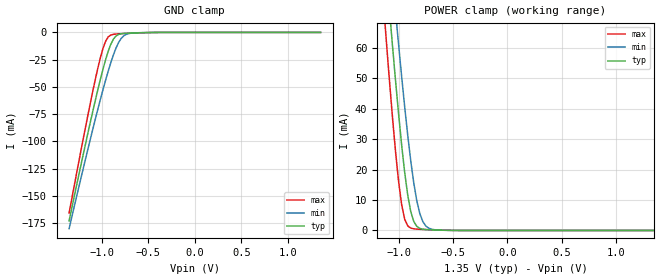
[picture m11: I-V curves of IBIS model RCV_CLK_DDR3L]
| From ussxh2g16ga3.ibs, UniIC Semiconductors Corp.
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|   Model RCV_CLK_DDR3L
[Model] RCV_CLK_DDR3L
Model_type Input
Vinl =  0.540V
Vinh =  0.810V
C_comp   0.694pF   0.694pF   0.694pF
[Model Spec]
Vinh   0.810V   0.776V   0.860V
Vinl   0.540V   0.506V   0.590V
[Temperature Range]   25.000   95.000   -40.000
[Voltage Range]   1.350V   1.283V   1.450V
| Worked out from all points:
|   GND clamp passes 1 mA (typ) near -0.77 V on its own axis
|   POWER clamp passes 1 mA (typ) near -0.82 V on its own axis
[GND_clamp]
|Voltage   I(typ)   I(min)   I(max)
-1.35V    -172.8mA   -179.9mA   -165.6mA
-1.126V   -83.84mA   -99.28mA   -66.45mA
-1.042V   -52.74mA   -70.63mA   -32.99mA
-986mV    -33.67mA   -52.44mA   -14.65mA
-958mV    -25.01mA   -43.77mA   -8.111mA
-930mV    -17.28mA   -35.47mA   -4.148mA
-874mV    -6.14mA    -20.55mA   -1.757mA
-818mV    -1.855mA   -9.196mA   -1.324mA
-762mV    -945.5uA   -3.027mA   -1.066mA
-678mV    -590.3uA   -656.8uA   -726.4uA
-510mV    -182.2uA   -145.1uA   -204.7uA
1.35V     0A         0A         0A
[POWER_clamp]
|Voltage   I(typ)   I(min)   I(max)
-1.35V    193.8mA    208.2mA    178.6mA
-1.142V   96.99mA    117.7mA    74.78mA
-1.114V   84.55mA    105.9mA    61.67mA
-1.086V   72.36mA    94.36mA    48.99mA
-1.058V   60.5mA     82.98mA    36.93mA
-1.03V    49.04mA    71.84mA    25.78mA
-1.002V   38.16mA    61.01mA    16.03mA
-946mV    19.05mA    40.6mA     3.667mA
-890mV    6.184mA    22.84mA    783.6uA
-806mV    668.6uA    5.465mA    387.3uA
-694mV    183.6uA    385.8uA    217.6uA
1.35V     0A         0A         0A
